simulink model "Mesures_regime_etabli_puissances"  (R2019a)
settings: Solver=ode45  StartTime=0.0  StopTime=1  RelTol=1e-3  EnableMultiTasking=on
InitFcn:
  | Fo=0.0135;
  | R=0.4;
  | L=0.0002;
  | Ki=0.11;
  | Ke=0.22;
  | Co=0,35288157;
  | Jmot=0.002;
libraries: powerlib x15, simulink x1

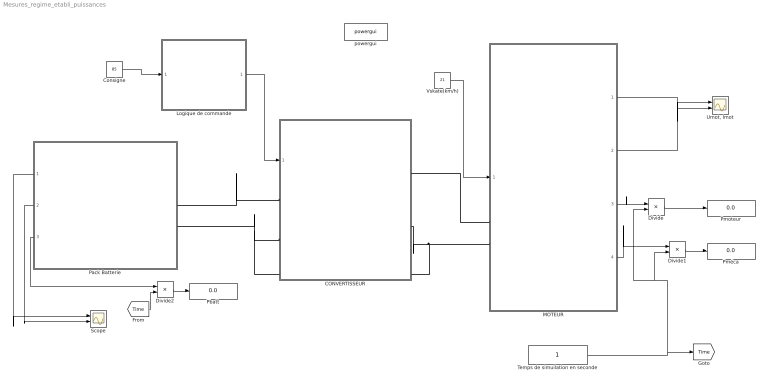
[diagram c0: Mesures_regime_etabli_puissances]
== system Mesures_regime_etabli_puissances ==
  CONVERTISSEUR : Subsystem
  Consigne : Constant  Value=85
  Divide : Product  Inputs=*/
  Divide1 : Product  Inputs=*/
  Divide2 : Product  Inputs=*/
  Logique de commande : Subsystem
  MOTEUR : Subsystem
  Pack Batterie : Subsystem
  Pbatt : Display
  Pmoteur : Display
  Pméca : Display
  Scope : Scope  NumInputPorts=2
  Temps de simuilation en seconde : Constant
  "Umot, Imot" : Scope  NumInputPorts=2
  Vskate(km/h) : Constant  Value=21
  powergui : powerlib/powergui  SimulationMode=Continuous  SampleTime=5e-9  frequency=60  Iterations=50  frequencyindice=0  Pbase=100e6  ErrMax=1e-4  UnitsV=kV  UnitsW=MW  buscounter=0  FunctionMessages=off  echomessages=off  EnableUseOfTLC=off  CurrentSourceSwitches=on  DisableSnubberDevices=off  DisableRonSwitches=off  DisableVfSwitches=off  DisplayEquations=off  AutomaticDiscreteSolvers=off  SolverType=Tustin  Interpol=off  ExternalGateDelay=off  methode=off  Ts=0  x0status=blocks  SPID=off  SwTol=0  HookPort=off  NonlinearTolerance=0  nMaxIteration=15  ContinueOnMaxIteration=off  RestoreLinks=warning  ResistiveCurrentMeasurement=off  Frange=[0:2:500]  Ylog=off  Xlog=on  ShowGrid=off  save=off  variable=ZData  structure=0  ZoomFFT=on  StartTime=0.0  cycles=1  DisplayStyle=1  fundamental=60  FreqAxis=off  MaxFrequency=1000  frequencyindicesteady=1  RmsSteady=1  display=off
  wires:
  Vskate(km/h)/1 -> MOTEUR/1(Vskate(km/h))
  MOTEUR/1(Umot_mesure) -> "Umot, Imot"/1
  MOTEUR/2(Imot_mesure) -> "Umot, Imot"/2
  Consigne/1 -> Logique de commande/1(Rapport cyclique)
  Divide/1 -> Pmoteur/1
  MOTEUR/3(Pelec*Temps simule) -> Divide/1
  Divide1/1 -> Pméca/1
  MOTEUR/4(Pmeca*Temps simule) -> Divide1/1
  Temps de simuilation en seconde/1 -> [Time], Divide/2, Divide1/2
  Logique de commande/1(Commande T) -> CONVERTISSEUR/1(In1)
  Pack Batterie/1(Ubatt) -> Scope/1
  Pack Batterie/2(Ibatt) -> Scope/2
  [Time] -> Divide2/2
  Pack Batterie/3(Pbatt) -> Divide2/1
  Divide2/1 -> Pbatt/1
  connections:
  MOTEUR/LConn2 -- CONVERTISSEUR/RConn2 -- Pack Batterie/LConn2 -- CONVERTISSEUR/LConn2
  CONVERTISSEUR/LConn1 -- Pack Batterie/LConn1
  MOTEUR/LConn1 -- CONVERTISSEUR/RConn1

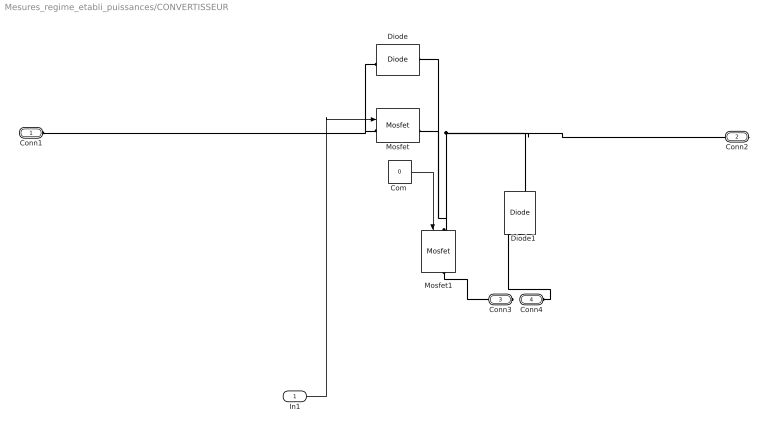
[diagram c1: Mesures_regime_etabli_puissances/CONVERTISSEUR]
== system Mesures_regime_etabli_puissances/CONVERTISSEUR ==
  In1 : Inport
  "Com " : Constant  Value=0
  Diode : powerlib/Power Electronics/Diode  Ron=0.001  Lon=0  Vf=0.8  IC=0  UseSnubber=off  Rs=500  Cs=250e-9  Measurements=on
  Diode1 : powerlib/Power Electronics/Diode  Ron=0.001  Lon=0  Vf=0.8  IC=0  UseSnubber=off  Rs=500  Cs=250e-9  Measurements=on
  Mosfet : powerlib/Power Electronics/Mosfet  Ron=0.1  Lon=0  Rd=0.001  Vfd=0.8  IC=0  Rs=1e5  Cs=inf  Measurements=on
  Mosfet1 : powerlib/Power Electronics/Mosfet  Ron=0.1  Lon=0  Rd=0.001  Vfd=0.8  IC=0  Rs=1e5  Cs=inf  Measurements=on
  Conn1 : PMIOPort  Side=Left
  Conn2 : PMIOPort  Port=2  Side=Right
  Conn3 : PMIOPort  Port=3  Side=Right
  Conn4 : PMIOPort  Port=4  Side=Left
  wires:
  "Com "/1 -> Mosfet1/1
  In1/1 -> Mosfet/1
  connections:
  Mosfet1/LConn1 -- Conn2/RConn1 -- Diode1/RConn1 -- Mosfet/RConn1 -- Diode/LConn1
  Diode/RConn1 -- Conn1/RConn1 -- Mosfet/LConn1
  Mosfet1/RConn1 -- Conn3/RConn1
  Conn4/RConn1 -- Diode1/LConn1

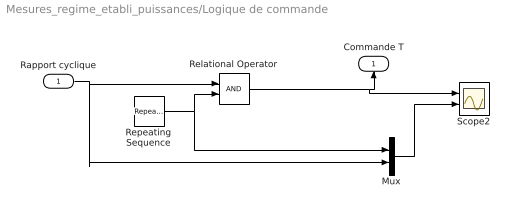
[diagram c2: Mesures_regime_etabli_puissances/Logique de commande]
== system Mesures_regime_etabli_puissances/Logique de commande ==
  Rapport cyclique : Inport
  Mux : Mux  Inputs=2
  Relational Operator : RelationalOperator  OutDataTypeStr=boolean
  Repeating Sequence : simulink/Sources/Repeating Sequence  rep_seq_t=[0 1624e-6]  rep_seq_y=[0 100]
  Scope2 : Scope  NumInputPorts=2
  Commande T : Outport
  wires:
  Repeating Sequence/1 -> Relational Operator/2, Mux/1
  Rapport cyclique/1 -> Mux/2, Relational Operator/1
  Relational Operator/1 -> Scope2/1, Commande T/1
  Mux/1 -> Scope2/2

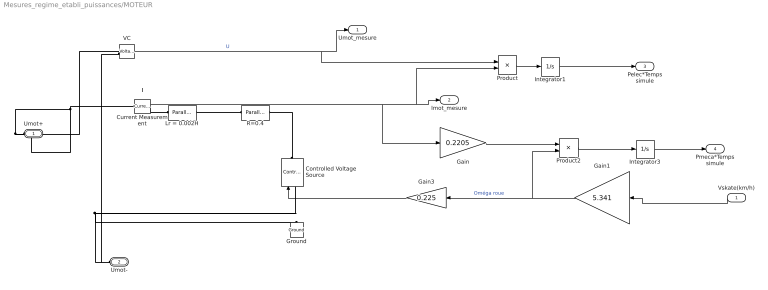
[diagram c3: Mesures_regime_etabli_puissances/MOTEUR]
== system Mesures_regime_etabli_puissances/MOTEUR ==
  note: I
  Vskate(km/h) : Inport
  Controlled Voltage Source : powerlib/Electrical Sources/Controlled Voltage Source  Initialize=on  Source_Type=DC  Amplitude=0  Phase=0  Frequency=0  Measurements=None
  Current Measurement : powerlib/Measurements/Current Measurement  PhasorSimulation=off  OutputType=Complex  PSBequivalent=0
  Gain : Gain  Gain=0.2205
  Gain1 : Gain  Gain=5.341
  Gain3 : Gain  Gain=0.225
  Ground : powerlib/Elements/Ground  LConnTagsString=a
  Integrator1 : Integrator
  Integrator3 : Integrator
  Lr = 0.002H : powerlib/Elements/Parallel RLC Branch  LConnTagsString=a  RConnTagsString=__new0  BranchType=L  Resistance=[]  Inductance=L  SetiL0=on  InitialCurrent=0  Capacitance=[]  Setx0=off  InitialVoltage=0  Measurements=None
  Product : Product
  Product2 : Product
  R=0.4 : powerlib/Elements/Parallel RLC Branch  LConnTagsString=a  RConnTagsString=__new0  BranchType=R  Resistance=[R]  Inductance=0.02e-6  SetiL0=on  InitialCurrent=0  Capacitance=[]  Setx0=off  InitialVoltage=0  Measurements=None
  VC : powerlib/Measurements/Voltage Measurement  Tag=PoWeRsYsTeMmEaSuReMeNt  PhasorSimulation=off  OutputType=Magnitude  PSBequivalent=0
  Umot+ : PMIOPort  Side=Left
  Umot- : PMIOPort  Port=2  Side=Left
  Umot_mesure : Outport
  Imot_mesure : Outport  Port=2
  Pelec*Temps simule : Outport  Port=3
  Pmeca*Temps simule : Outport  Port=4
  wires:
  Gain3/1 -> Controlled Voltage Source/1
  Gain1/1 -> Gain3/1, Product2/2  "Oméga roue"
  VC/1 -> Umot_mesure/1, Product/1  "U"
  Current Measurement/1 -> Imot_mesure/1, Product/2, Gain/1
  Vskate(km/h)/1 -> Gain1/1
  Product/1 -> Integrator1/1
  Integrator1/1 -> Pelec*Temps simule/1
  Gain/1 -> Product2/1
  Product2/1 -> Integrator3/1
  Integrator3/1 -> Pmeca*Temps simule/1
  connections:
  Umot-/RConn1 -- Controlled Voltage Source/LConn1 -- Ground/LConn1 -- VC/LConn2
  Controlled Voltage Source/RConn1 -- R=0.4/RConn1
  Umot+/RConn1 -- VC/LConn1 -- Current Measurement/LConn1
  Current Measurement/RConn1 -- Lr = 0.002H/LConn1
  Lr = 0.002H/RConn1 -- R=0.4/LConn1

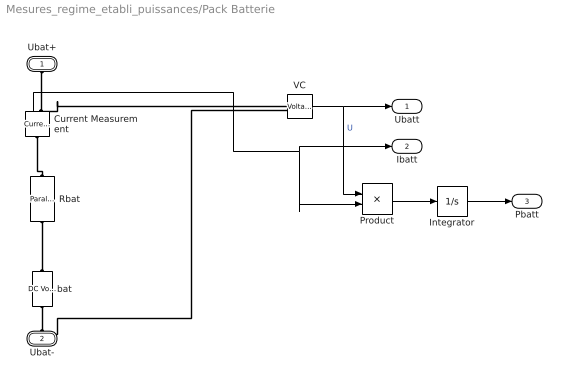
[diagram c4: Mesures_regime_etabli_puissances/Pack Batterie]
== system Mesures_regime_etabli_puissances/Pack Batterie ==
  Current Measurement : powerlib/Measurements/Current Measurement  PhasorSimulation=off  OutputType=Complex  PSBequivalent=0
  Integrator : Integrator
  Product : Product
  Rbat : powerlib/Elements/Parallel RLC Branch  LConnTagsString=a  RConnTagsString=__new0  BranchType=R  Resistance=[0.1]  Inductance=0.02e-6  SetiL0=on  InitialCurrent=0  Capacitance=[]  Setx0=off  InitialVoltage=0  Measurements=None
  VC : powerlib/Measurements/Voltage Measurement  Tag=PoWeRsYsTeMmEaSuReMeNt  PhasorSimulation=off  OutputType=Magnitude  PSBequivalent=0
  bat : powerlib/Electrical Sources/DC Voltage Source  Description=source block  Amplitude=40  Measurements=None
  Ubat+ : PMIOPort  Side=Left
  Ubat- : PMIOPort  Port=2  Side=Left
  Ubatt : Outport
  Ibatt : Outport  Port=2
  Pbatt : Outport  Port=3
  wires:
  VC/1 -> Product/1, Ubatt/1  "U"
  Current Measurement/1 -> Product/2, Ibatt/1
  Product/1 -> Integrator/1
  Integrator/1 -> Pbatt/1
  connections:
  bat/RConn1 -- Rbat/RConn1
  Ubat-/RConn1 -- VC/LConn2 -- bat/LConn1
  Rbat/LConn1 -- Current Measurement/LConn1
  Current Measurement/RConn1 -- Ubat+/RConn1 -- VC/LConn1
